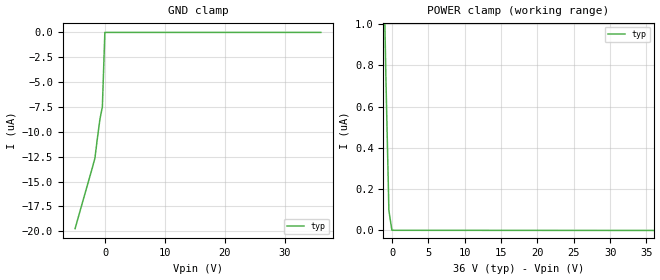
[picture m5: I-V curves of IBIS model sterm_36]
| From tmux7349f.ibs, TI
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| sterm_36
[Model]   sterm_36
Model_type   Terminator
|   typ   min   max
C_comp   1.598234e-12   NA   NA
[Voltage Range]   36   NA   NA
[Temperature Range]   27   NA   NA
[Power Clamp Reference]   36   NA   NA
[GND Clamp Reference]   0   NA   NA
[GND Clamp]
|   Voltage   I(typ)   I(min)   I(max)
-5V       -19.73uA   NA         NA
-1.687V   -12.64uA   NA         NA
-1.273V   -10.62uA   NA         NA
-858.6mV  -8.76uA    NA         NA
-444.4mV  -7.478uA   NA         NA
-30.3mV   -649.6pA   NA         NA
36V       814pA      NA         NA
[POWER Clamp]
|   Voltage   I(typ)   I(min)   I(max)
-5V       8.864uA    NA         NA
-1.273V   1.509uA    NA         NA
-858.6mV  744.9nA    NA         NA
-444.4mV  95.85nA    NA         NA
-30.3mV   831.7pA    NA         NA
36V       -362.2pA   NA         NA
